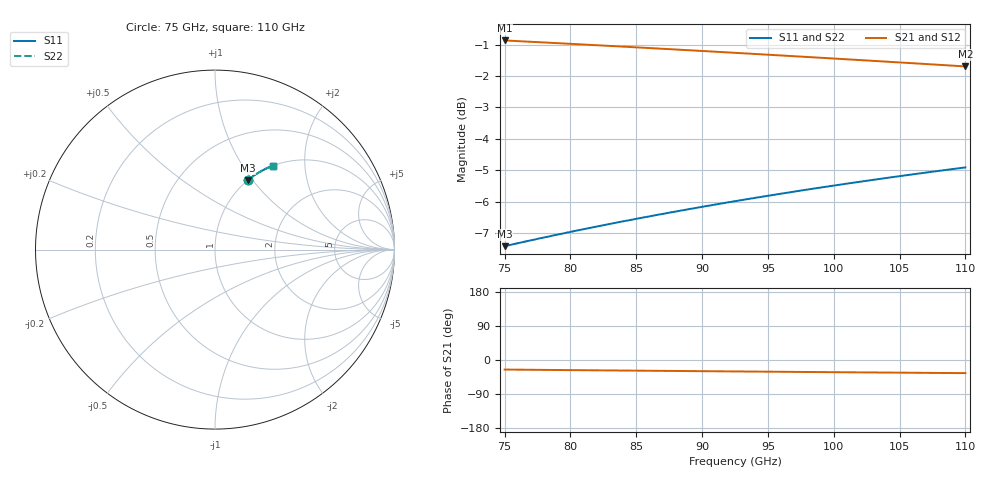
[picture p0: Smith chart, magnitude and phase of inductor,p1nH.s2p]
# HZ S RI R 50
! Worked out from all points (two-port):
!   101 points, 75 GHz to 110 GHz, reference 50 ohm
!   highest |S21| = -0.87 dB at 75 GHz (marker M1); lowest = -1.7 dB at 110 GHz (marker M2)
!   |S21| within 3 dB of the highest: start of sweep to end of sweep
!   lowest |S11| = -7.4 dB at 75 GHz (marker M3), VSWR 2.49, Z = 50 + j47.1 ohm
!   |S11| at or under -10 dB: nowhere
!   |S22| runs from -7.4 to -4.9 dB; largest |S21 - S12| = 0
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7.5e10  0.1817 0.3856  0.8183 -0.3856  0.8183 -0.3856  0.1817 0.3856
7.64e10  0.1873 0.3901  0.8127 -0.3901  0.8127 -0.3901  0.1873 0.3901
7.78e10  0.1929 0.3946  0.8071 -0.3946  0.8071 -0.3946  0.1929 0.3946
7.92e10  0.1985 0.3989  0.8015 -0.3989  0.8015 -0.3989  0.1985 0.3989
8.095e10  0.2055 0.4041  0.7945 -0.4041  0.7945 -0.4041  0.2055 0.4041
8.235e10  0.2112 0.4081  0.7888 -0.4081  0.7888 -0.4081  0.2112 0.4081
8.375e10  0.2169 0.4121  0.7831 -0.4121  0.7831 -0.4121  0.2169 0.4121
8.515e10  0.2225 0.416  0.7775 -0.416  0.7775 -0.416  0.2225 0.416
8.69e10  0.2297 0.4206  0.7703 -0.4206  0.7703 -0.4206  0.2297 0.4206
8.83e10  0.2354 0.4242  0.7646 -0.4242  0.7646 -0.4242  0.2354 0.4242
8.97e10  0.2411 0.4277  0.7589 -0.4277  0.7589 -0.4277  0.2411 0.4277
9.11e10  0.2468 0.4311  0.7532 -0.4311  0.7532 -0.4311  0.2468 0.4311
9.25e10  0.2525 0.4344  0.7475 -0.4344  0.7475 -0.4344  0.2525 0.4344
9.39e10  0.2582 0.4376  0.7418 -0.4376  0.7418 -0.4376  0.2582 0.4376
9.53e10  0.2639 0.4408  0.7361 -0.4408  0.7361 -0.4408  0.2639 0.4408
9.67e10  0.2696 0.4438  0.7304 -0.4438  0.7304 -0.4438  0.2696 0.4438
9.845e10  0.2767 0.4474  0.7233 -0.4474  0.7233 -0.4474  0.2767 0.4474
1.0125e11  0.2881 0.4529  0.7119 -0.4529  0.7119 -0.4529  0.2881 0.4529
1.0265e11  0.2938 0.4555  0.7062 -0.4555  0.7062 -0.4555  0.2938 0.4555
1.044e11  0.3008 0.4586  0.6992 -0.4586  0.6992 -0.4586  0.3008 0.4586
1.072e11  0.3121 0.4633  0.6879 -0.4633  0.6879 -0.4633  0.3121 0.4633
1.1e11  0.3233 0.4677  0.6767 -0.4677  0.6767 -0.4677  0.3233 0.4677
